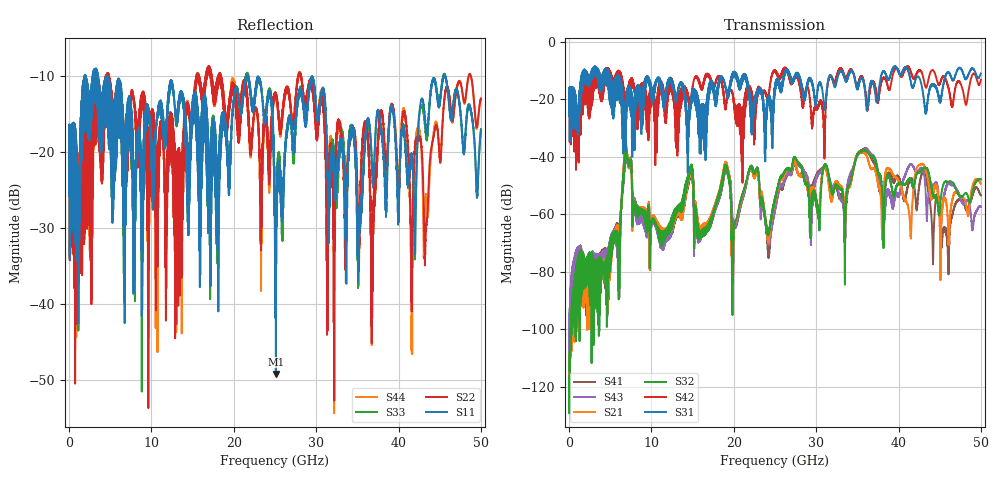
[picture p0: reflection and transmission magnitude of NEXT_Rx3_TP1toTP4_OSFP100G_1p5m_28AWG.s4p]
! Touchstone data
! Created: 27-Feb-2019 by IdEM 12 (12.1.0)
! COMMENTS
!  Created Wed Feb 27 09:43:39 2019
!  64 Port Network Data from SP1.SP block
!  freq  magS1_1  angS1_1  magS1_2  angS1_2  magS1_3  angS1_3  magS1_4  angS1_4
!  magS1_5  angS1_5  magS1_6  angS1_6  magS1_7  angS1_7  magS1_8  angS1_8
!  magS1_9  angS1_9  magS1_10  angS1_10  magS1_11  angS1_11  magS1_12  angS1_12
!  magS1_13  angS1_13  magS1_14  angS1_14  magS1_15  angS1_15  magS1_16  angS1_16
!  magS1_17  angS1_17  magS1_18  angS1_18  magS1_19  angS1_19  magS1_20  angS1_20
!  magS1_21  angS1_21  magS1_22  angS1_22  magS1_23  angS1_23  magS1_24  angS1_24
!  magS1_25  angS1_25  magS1_26  angS1_26  magS1_27  angS1_27  magS1_28  angS1_28
!  magS1_29  angS1_29  magS1_30  angS1_30  magS1_31  angS1_31  magS1_32  angS1_32
!  magS1_33  angS1_33  magS1_34  angS1_34  magS1_35  angS1_35  magS1_36  angS1_36
!  magS1_37  angS1_37  magS1_38  angS1_38  magS1_39  angS1_39  magS1_40  angS1_40
!  magS1_41  angS1_41  magS1_42  angS1_42  magS1_43  angS1_43  magS1_44  angS1_44
!  magS1_45  angS1_45  magS1_46  angS1_46  magS1_47  angS1_47  magS1_48  angS1_48
!  magS1_49  angS1_49  magS1_50  angS1_50  magS1_51  angS1_51  magS1_52  angS1_52
!  magS1_53  angS1_53  magS1_54  angS1_54  magS1_55  angS1_55  magS1_56  angS1_56
!  magS1_57  angS1_57  magS1_58  angS1_58  magS1_59  angS1_59  magS1_60  angS1_60
!  magS1_61  angS1_61  magS1_62  angS1_62  magS1_63  angS1_63  magS1_64  angS1_64
!  magS2_1  angS2_1  magS2_2  angS2_2  magS2_3  angS2_3  magS2_4  angS2_4
!  magS2_5  angS2_5  magS2_6  angS2_6  magS2_7  angS2_7  magS2_8  angS2_8
!  magS2_9  angS2_9  magS2_10  angS2_10  magS2_11  angS2_11  magS2_12  angS2_12
!  magS2_13  angS2_13  magS2_14  angS2_14  magS2_15  angS2_15  magS2_16  angS2_16
!  magS2_17  angS2_17  magS2_18  angS2_18  magS2_19  angS2_19  magS2_20  angS2_20
!  magS2_21  angS2_21  magS2_22  angS2_22  magS2_23  angS2_23  magS2_24  angS2_24
!  magS2_25  angS2_25  magS2_26  angS2_26  magS2_27  angS2_27  magS2_28  angS2_28
!  magS2_29  angS2_29  magS2_30  angS2_30  magS2_31  angS2_31  magS2_32  angS2_32
!  magS2_33  angS2_33  magS2_34  angS2_34  magS2_35  angS2_35  magS2_36  angS2_36
!  magS2_37  angS2_37  magS2_38  angS2_38  magS2_39  angS2_39  magS2_40  angS2_40
!  magS2_41  angS2_41  magS2_42  angS2_42  magS2_43  angS2_43  magS2_44  angS2_44
!  magS2_45  angS2_45  magS2_46  angS2_46  magS2_47  angS2_47  magS2_48  angS2_48
!  magS2_49  angS2_49  magS2_50  angS2_50  magS2_51  angS2_51  magS2_52  angS2_52
!  magS2_53  angS2_53  magS2_54  angS2_54  magS2_55  angS2_55  magS2_56  angS2_56
!  magS2_57  angS2_57  magS2_58  angS2_58  magS2_59  angS2_59  magS2_60  angS2_60
!  magS2_61  angS2_61  magS2_62  angS2_62  magS2_63  angS2_63  magS2_64  angS2_64
!  magS3_1  angS3_1  magS3_2  angS3_2  magS3_3  angS3_3  magS3_4  angS3_4
!  magS3_5  angS3_5  magS3_6  angS3_6  magS3_7  angS3_7  magS3_8  angS3_8
!  magS3_9  angS3_9  magS3_10  angS3_10  magS3_11  angS3_11  magS3_12  angS3_12
!  magS3_13  angS3_13  magS3_14  angS3_14  magS3_15  angS3_15  magS3_16  angS3_16
!  magS3_17  angS3_17  magS3_18  angS3_18  magS3_19  angS3_19  magS3_20  angS3_20
!  magS3_21  angS3_21  magS3_22  angS3_22  magS3_23  angS3_23  magS3_24  angS3_24
!  magS3_25  angS3_25  magS3_26  angS3_26  magS3_27  angS3_27  magS3_28  angS3_28
!  magS3_29  angS3_29  magS3_30  angS3_30  magS3_31  angS3_31  magS3_32  angS3_32
!  magS3_33  angS3_33  magS3_34  angS3_34  magS3_35  angS3_35  magS3_36  angS3_36
!  magS3_37  angS3_37  magS3_38  angS3_38  magS3_39  angS3_39  magS3_40  angS3_40
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# Hz S MA R 50
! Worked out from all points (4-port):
!   5000 points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, 10 MHz to 50 GHz, reference 50 ohm
!   strongest paths, dB at 10 MHz, 12.51 GHz, 25.01 GHz, 37.51 GHz, 50 GHz:
!     S31: -19.6, -14.0, -15.9, -19.1, -11.0
!     S42: -19.6, -16.1, -10.2, -20.9, -13.2
!     S32: -117.2, -64.9, -54.8, -45.9, -47.9
!     S21: -119.5, -65.3, -55.4, -49.7, -49.3
!     S43: -111.4, -66.3, -57.9, -44.7, -57.4
!     S41: -112.1, -66.8, -58.0, -48.0, -53.5
!   lowest |S11| = -49.2 dB at 25.11 GHz (marker M1), VSWR 1.01, Z = 50.3 + j0.113 ohm
!   |S11| at or under -10 dB: 4.66 GHz to 21.51 GHz (16.85 GHz wide, 129 % of centre); 22.94 GHz to 45.47 GHz (22.53 GHz wide, 65.9 % of centre); 45.68 GHz to end of sweep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
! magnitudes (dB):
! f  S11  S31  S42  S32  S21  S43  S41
! 10 MHz  -19.2  -19.6  -19.6  -117.2  -119.5  -111.4  -112.1
! 4.69 GHz  -14.2  -14.5  -12.4  -89.0  -89.1  -77.2  -76.5
! 6.94 GHz  -17.5  -19.7  -19.8  -37.3  -35.7  -38.7  -37.0
! 11.28 GHz  -14.0  -15.8  -15.4  -71.1  -68.5  -71.7  -69.1
! 14.75 GHz  -21.0  -21.8  -21.3  -43.8  -44.8  -44.8  -45.8
! 25.11 GHz  -49.2  -14.8  -10.5  -53.5  -54.0  -56.4  -56.5
! 50 GHz  -17.1  -11.0  -13.2  -47.9  -49.3  -57.4  -53.5
